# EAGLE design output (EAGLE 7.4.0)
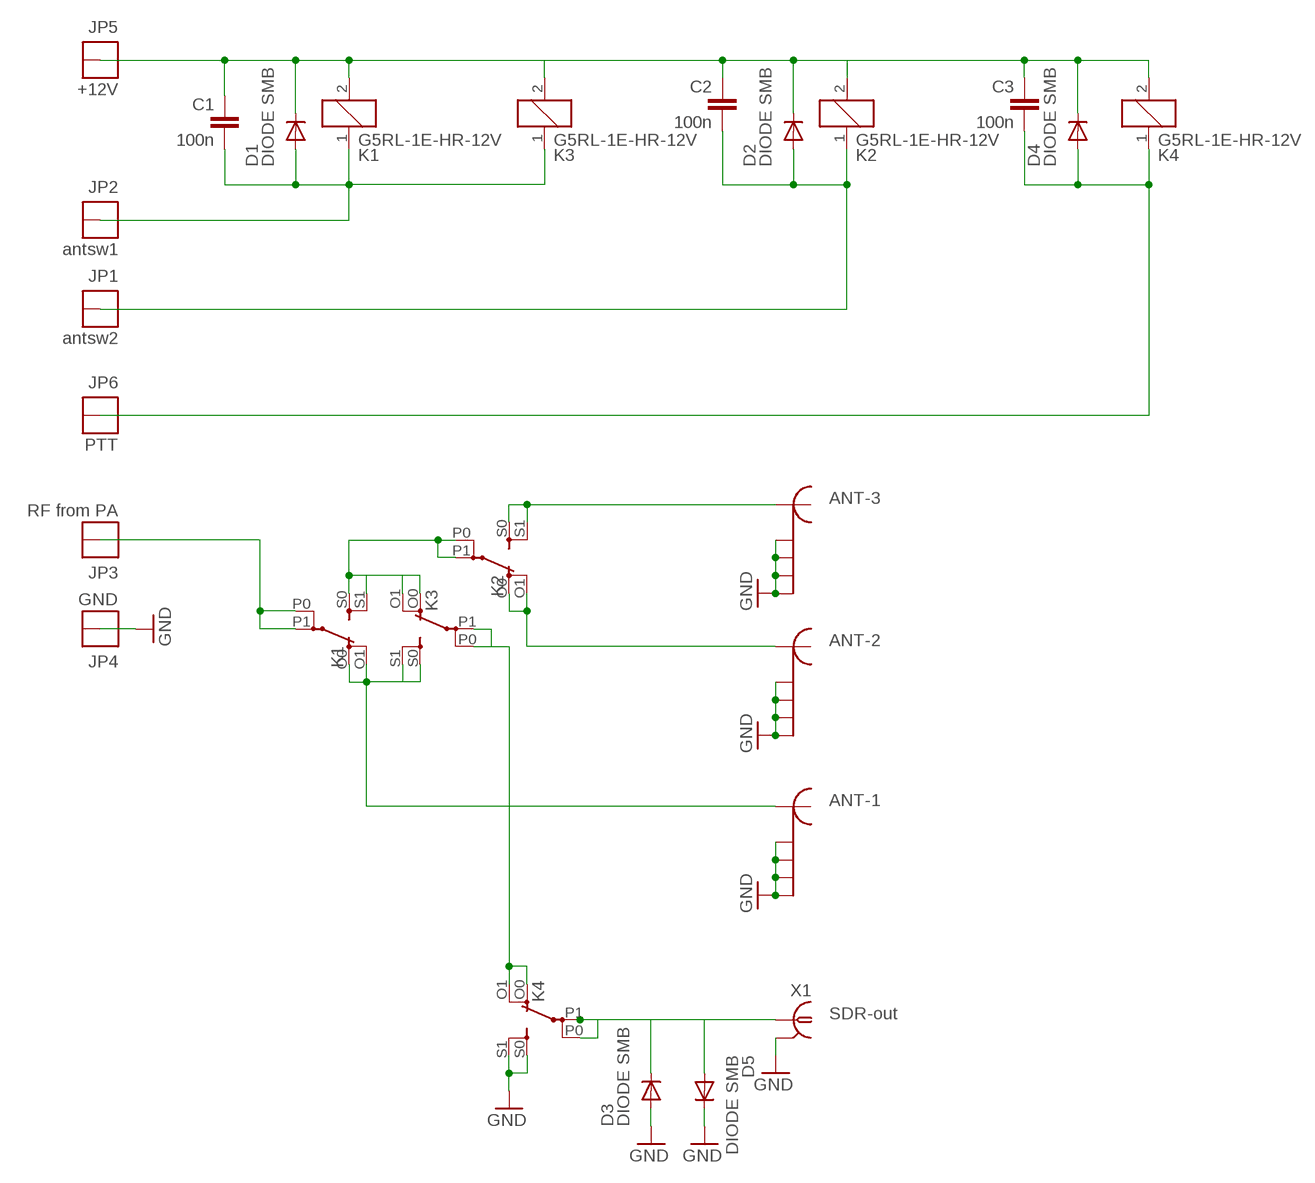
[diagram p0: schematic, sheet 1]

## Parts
C1  100n  C-EUC0805  [C0805]
C2  100n  C-EUC0805  [C0805]
C3  100n  C-EUC0805  [C0805]
CON1  PL_CONNECTOR  [PL_CONNECTOR]
CON2  PL_CONNECTOR  [PL_CONNECTOR]
CON3  PL_CONNECTOR  [PL_CONNECTOR]
D1  DIODE SMB  DIODE-MINIMELF  [MINIMELF]
D2  DIODE SMB  DIODE-MINIMELF  [MINIMELF]
D3  DIODE SMB  DIODE-MINIMELF  [MINIMELF]
D4  DIODE SMB  DIODE-MINIMELF  [MINIMELF]
D5  DIODE SMB  DIODE-MINIMELF  [MINIMELF]
JP1  antsw2  THICKPINSQUARE  [THICKPIN]
JP2  antsw1  THICKPINSQUARE  [THICKPIN]
JP3  RF from PA  THICKPINSQUARE  [THICKPIN]
JP4  GND  THICKPINSQUARE  [THICKPIN]
JP5  +12V  THICKPINSQUARE  [THICKPIN]
JP6  PTT  THICKPINSQUARE  [THICKPIN]
K1  G5RL-1E-HR-12V  G2RE  [G2RE]
K2  G5RL-1E-HR-12V  G2RE  [G2RE]
K3  G5RL-1E-HR-12V  G2RE  [G2RE]
K4  G5RL-1E-HR-12V  G2RE  [G2RE]
X1  A1944-50  [A1944]

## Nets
A1: C1.2 D1.A JP2.1 K1.1 K3.1
A2: C2.2 D2.A JP1.1 K2.1
GND: CON1.G1 CON1.G2 CON1.G3 CON1.G4 CON2.G1 CON2.G2 CON2.G3 CON2.G4 CON3.G1 CON3.G2 CON3.G3 CON3.G4 D3.A D5.C JP4.1 K4.S0(2:S) K4.S1(2:S) X1.2 X1.3 X1.4 X1.5
N$3: JP3.1 K1.P0(2:P) K1.P1(2:P)
N$4: K1.S0(2:S) K1.S1(2:S) K2.P0(2:P) K2.P1(2:P) K3.O0(2:O) K3.O1(2:O)
N$5: C1.1 C2.1 C3.1 D1.C D2.C D4.C JP5.1 K1.2 K2.2 K3.2 K4.2
N$6: D3.C D5.A K4.P0(2:P) K4.P1(2:P) X1.1
N$7: CON3.M K1.O0(2:O) K1.O1(2:O) K3.S0(2:S) K3.S1(2:S)
N$8: CON1.M K2.S0(2:S) K2.S1(2:S)
N$9: CON2.M K2.O0(2:O) K2.O1(2:O)
N$12: K3.P0(2:P) K3.P1(2:P) K4.O0(2:O) K4.O1(2:O)
PTT: C3.2 D4.A JP6.1 K4.1

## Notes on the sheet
- ANT-3
- ANT-2
- ANT-1
- SDR-out

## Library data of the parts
C1-C3 = rcl:C-EU: CAPACITOR, European symbol
CON1-CON3 = km:PL_CONNECTOR
D1-D5 = diode:DIODE-: DIODE
JP1-JP6 = km:THICKPIN
K1-K4 = relay:G2RE: RELAY 1 x switch, high current, Omron; OC_FARNELL: unknown; OC_NEWARK: unknown
X1 = con-coax:A1944-50: BNC CONNECTOR 50 Ohm; OC_FARNELL: unknown; OC_NEWARK: unknown

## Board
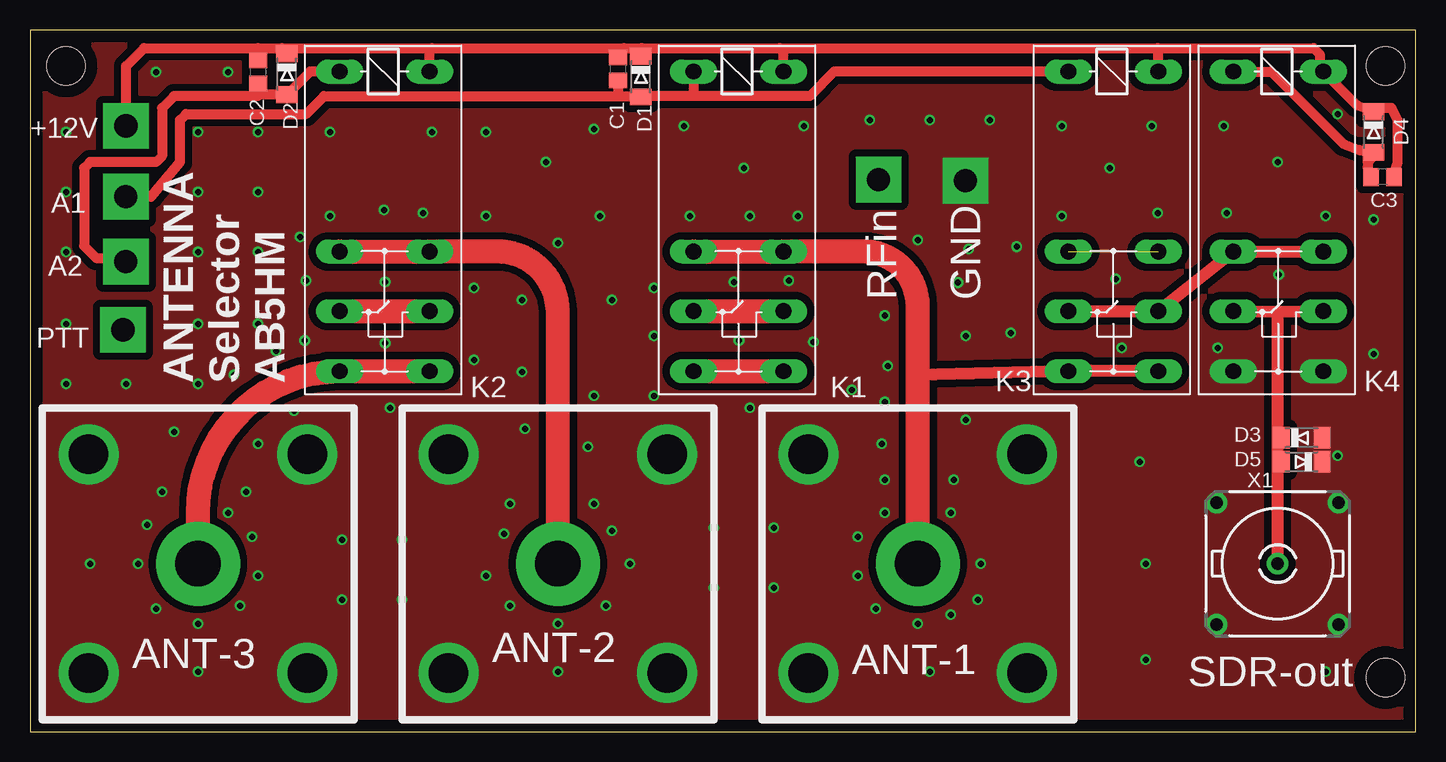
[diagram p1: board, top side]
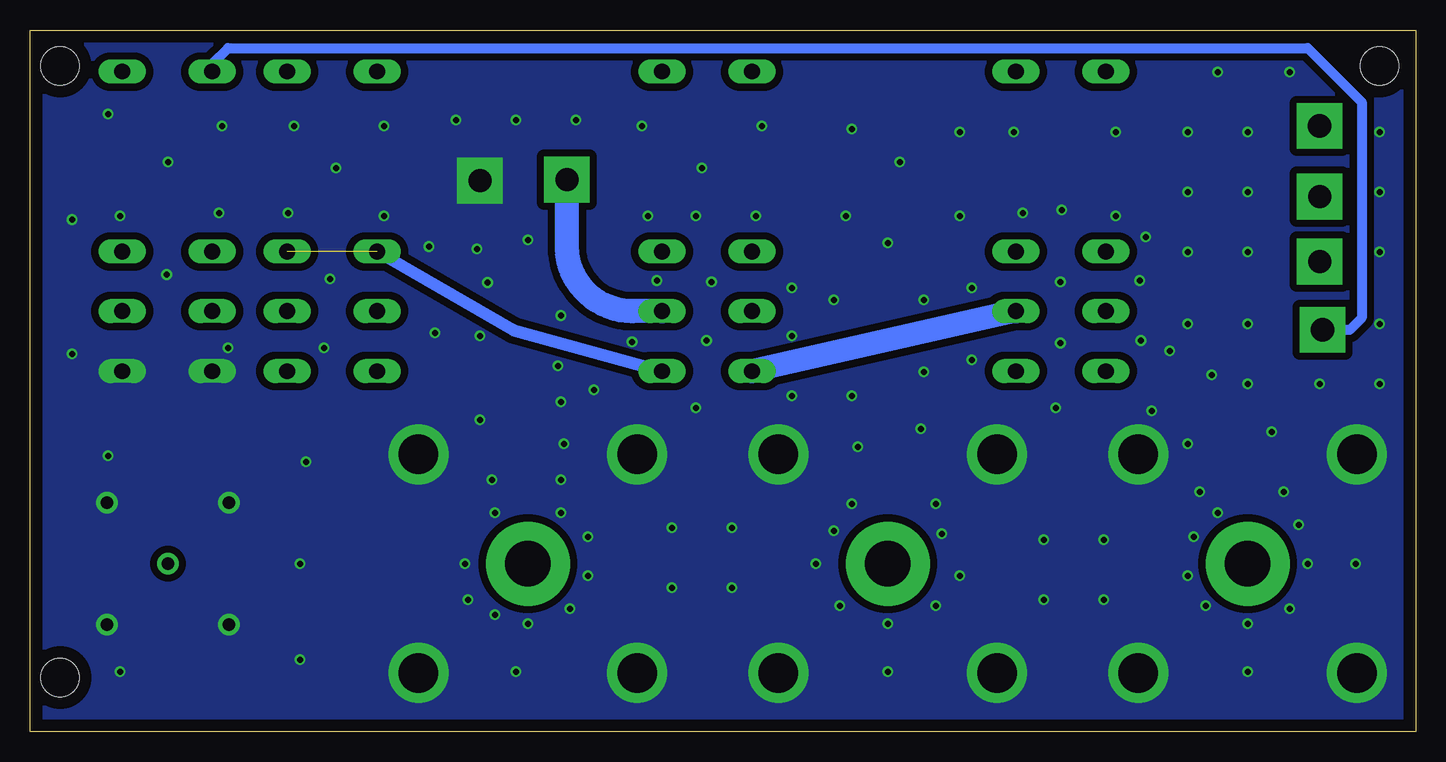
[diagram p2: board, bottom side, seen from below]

Size 115.5 x 58.5 mm. Coordinates in mm from the lower left corner, seen from the top.
Outline: 0,0 115.5,0 115.5,58.5 0,58.5 0,0
Copper layers (1*16): Top 0.035mm / dielectric 1.5mm / Bottom 0.035mm
Design rules "default *": minimum track width 10mil, minimum drill 0.3mm, track to track 8mil, track to pad 8mil, pad to pad 8mil, via to via 8mil, smd to smd 8mil, copper to edge 40mil, drill to drill 8mil, minimum pad ring 10mil, minimum via ring 8mil, stop-mask expansion 4mil, vias tented up to drill 0.51mm, thermal gap 10mil
Holes 3.2 mm at 3,55.5 113,55.5 113,4.5

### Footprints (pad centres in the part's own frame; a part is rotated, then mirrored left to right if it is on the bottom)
C0805 = smd 1.3 x 1.5: 1 -0.95,0; 2 0.95,0
PL_CONNECTOR = drill 3.3 pad 5: G1 -9.12,9.12; G2 9.12,9.12; G3 -9.12,-9.12; G4 9.12,-9.12 | drill 3.8 pad 7: M 0,0
MINIMELF = smd 1.4 x 1.8: A 1.7,0; C -1.7,0
THICKPIN = drill 1.93 pad 3.81 square: 1 0,0
G2RE = drill 1.321 long: 1 -2.54,-3.683; 2 -2.54,3.81; O0 12.471,-3.683; O1 12.471,3.81; P0 17.45,-3.683; P1 17.45,3.81; S0 22.454,-3.683; S1 22.454,3.81
A1944 = drill 1.016 pad 1.778: 1 0,0; 2 5.08,5.08; 3 -5.08,5.08; 4 -5.08,-5.08; 5 5.08,-5.08

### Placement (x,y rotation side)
C1  49,55.25 270 top
C2  19,55 270 top
C3  112.75,46.25 180 top
CON1  14,14 0 top
CON2  44,14 0 top
CON3  74,14 0 top
D1  50.92,54.61 270 top
D2  21.42,54.81 270 top
D3  106,24.5 0 top
D4  112,50 270 top
D5  106,22.5 180 top
JP1  7.99,39.18 90 top
JP2  7.99,44.6 90 top
JP3  70.74,46.02 90 top
JP4  77.99,45.94 90 top
JP5  8,50.5 0 top
JP6  7.75,33.5 0 top
K1  59,52.5 270 top
K2  29.5,52.5 270 top
K3  90.25,52.5 270 top
K4  104,52.5 270 top
X1  104,14 0 top

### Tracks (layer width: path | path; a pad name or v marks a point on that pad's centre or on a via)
A1
  Top 0.813: K3.1 67.04,55.04 65,53 55.5,53 | 55.5,53 51.33,53 | 51.33,53 D1.A | JP2.1 10.1,44.6 12.5,47.5 12.5,51 13,51.5 23,51.5 24.5,53 49,53 | 49,53 51.33,53 | C1.2 49,53 | K1.1 55.32,53.18 55.5,53
A2
  Top 0.813: K2.1 23.35,55.04 D2.A 19.11,53.11 | 19.11,53.11 19,53 12,53 11,52 11,48 10.5,47.5 5,47.5 4.5,47 4.5,40.5 5.5,39.5 7.81,39.5 JP1.1 | C2.2 19,53.22 19.11,53.11
GND  (via drill 0.5)
  other vias: 3,50 3,45 3,40 3,34 3,29 33.5,50 90,47 104,47.5 59.5,47 8,29 14,50 14,45 14,40 14,34 14,29 19,50 19,45 19,40 19,34 26,16 26,11 31,16 31,11 57,17 57,12 62,17 62,12 109,51.5 86,50.5 75,51 99.5,50.5 37,37 37,31 41,36 41,30 38,50 92.5,22.5 47.5,43 52,37 48.5,36 47,28 52,33 52,28 54.5,50.5 60,43 64.5,50.5 64,43 80,51 70,51 109,23 99.75,43.25 74,41 93.5,50.5 108,43 86,43 25,43 29.5,43.5 25,50 38,43 82.25,40.45 68.5,28.5 71,24 108,5 75,5 44,5 14,5 5,14 47,19 40,19 18,20 11,20 12,25 30,27 60,27 99,32 93,14 91,32 112,31.5 78.25,40.25 94,43.25 77.35,37.45 78,33 43,47.5 78,26 77,21 93,6 69,13 74,9 79,11 50,14 38,13 44,9 19,13 9,14 14,9 19,24 16.5,55 10.5,55 58.7,37.5 59.1,32.6 65.3,32.5 63.25,37.6 29.6,37.5 29.6,32.4 22.9,32.6 23,37.6 104.1,38.1 71.25,34.7 112,42.7 41.25,25.25 71.25,27.5 71.25,21 71.5,30.5 81.75,33.25 55,43 44,40.75 32.75,43.25 22.5,41.25 46.5,23.75 90.5,37.75 47,50.25 20.5,31.75 17,29.75 22,26.75 9.75,17.25 18.5,16.25 17.5,10.5 10.5,10.25 39.5,16.5 40,10.5 48,10.5 48.5,16.75 69,16.25 70.5,10.25 76.75,9.75 79.25,14 76.75,18.25 71.25,18.25 16.5,18.25
  pour Bottom (isolate 0.61, no thermals): 0.5,58 114.5,58 114.5,1 0.5,1
  pour Top (isolate 0.61, no thermals): 0.75,57.75 114.75,57.75 114.75,0.75 0.75,0.75
N$3
  Top 2: K1.P0 K1.P1
  Bottom 2: K1.P1 65.3,35.05 arc90 70.75,40.5 JP3.1
N$4  (1 unrouted)
  Top 2: K2.P0 K2.P1 | K1.S0 K1.S1
  Bottom 1.016: K3.O0 75.25,33.5 K1.S1
  Bottom 2: K2.P1 K1.S0
N$5
  Top 0.813: JP5.1 8,55.5 9.5,57 19,57 | 19,57 21,57 | 21,57 33.5,57 | 33.5,57 49.5,57 | 49.5,57 51,57 | 51,57 62.5,57 | 62.5,57 94,57 | 94,57 107,57 107.5,56.5 107.5,55.23 | 94,57 94.06,56.94 K3.2 | K1.2 62.81,56.69 62.5,57 | K2.2 33.31,56.81 33.5,57 | C1.1 49,56.5 49.5,57 | D1.C 50.92,56.92 51,57 | D2.C 21.42,56.58 21,57 | C2.1 19,57 | K4.2 110.65,52.2 D4.C 112.7,52 113.5,52 114,51 114,47.5 113.75,46.75 C3.1
  Top 1.016: 107.5,55.23 K4.2
N$6
  Top 0.406: D3.C 104,24 | D5.A 104,22
  Top 1.016: X1.1 104,22 104,24 104,35 | 104,35 K4.P0 | K4.P1 104,35
N$7
  Top 1.016: K3.S1 K3.S0 74,29.75
  Top 2: K1.O0 K1.O1 69.47,40.03 arc-90 74,35.5 74,29.75 CON3.M
N$8
  Top 2: CON1.M 14,18.23 arc-90 K2.S0 K2.S1
N$9
  Top 2: CON2.M 44,35 arc90 38.97,40.03 K2.O1 K2.O0
N$12
  Top 1.016: K3.P0 K3.P1 K4.O0 K4.O1
PTT
  Top 0.813: K4.1 103.46,55.04 109.5,49 110.8,48.5 D4.A 111.8,47.8 111.5,47.5 111.5,47.05 C3.2
  Bottom 0.813: K4.1 100.32,55.68 99,57 9,57 4.5,52.5 4.5,34.5 5.5,33.5 JP6.1

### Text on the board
tNames: +12V | A1 | A2 | RFin | GND | PTT | ANTENNA / Selector / AB5HM | ANT-2 | ANT-3 | ANT-1 | SDR-out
